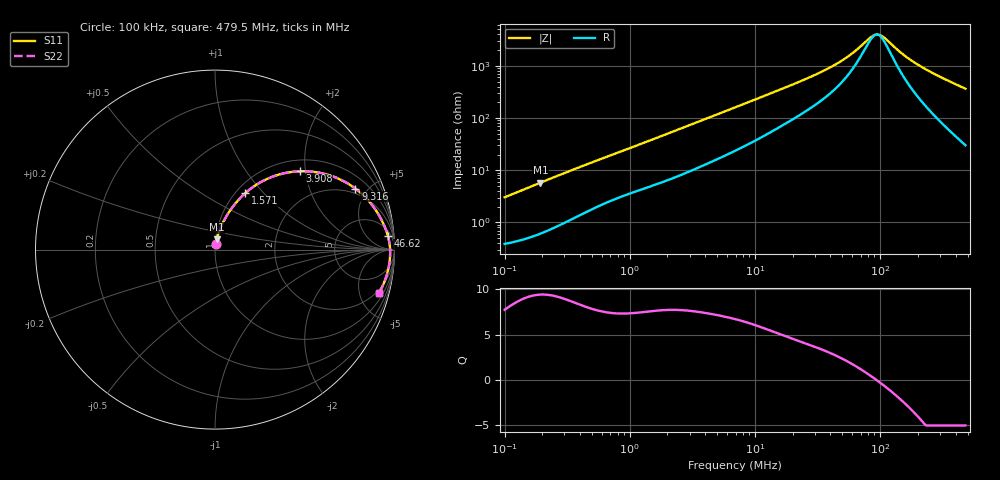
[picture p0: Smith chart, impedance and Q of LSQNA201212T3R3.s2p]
! LSQNA201212T3R3  S-PARAMETER MODEL  ( General Type )
! Model Generated by TAIYO YUDEN Corporation (http://www.ty-top.com)
! Version 2.0
! TAIYO YUDEN Control No. 100810NF25SB-FKC
! Copyright(c) 2007 TAIYO YUDEN CO.,LTD. All Rights Reserved.
! Product Description (link to TY-COMPAS)
! https://ds.yuden.co.jp/TYCOMPAS/or/detail?pn=LSQNA201212T3R3M&u=M
! Products Name : Inductors
! Characteristics :
!  Inductance : 3.3 uH , SRF(min) : 55 MHz , DC Resistance(max) : 0.39 Ohm
!  Rated Current : Saturation :330 mA , Temp Rise : 650 mA (40 degC)
!  Case Size : 2.0 x 1.25 / 0.079 x 0.049 [mm/inch] , Thickness : 1.25 / 0.049 [mm/inch]
!  (Conditions: Temperature = 25 degC , DC Bias Current/Voltage = 0A / 0V)
! External Node Assignments :
!  1  o---GGG---o  2
! GND o---------o GND
! Frequency Range : 0.1MHz  -  479.524407MHz  [ 402 STEP ]
# MHz S RI R 50
! Freq[MHz].  S11 Real  S11 Imag  S21 Real  S21 Imag  S12 Real  S12 Imag  S22 Real  S22 Imag
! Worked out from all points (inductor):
!   401 points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, 100 kHz to 479.5 MHz, reference 50 ohm
!   read as one part in series: L = 4.77 uH near 104.3 kHz
!   highest Q = 9.43 at 192.9 kHz (marker M1), where L = 4.73 uH
!   self-resonance near 93.8 MHz
!   S11 on the Smith chart (normalised r, x): 100 kHz: 1.01, +0.06; 1.571 MHz: 1.10, +0.80; 3.908 MHz: 1.25, +1.86; 9.316 MHz: 1.67, +4.17; 46.62 MHz: 9, +22; 479.5 MHz: 1.60, -7.30
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0.1  0.00475 0.0298  0.9952 -0.0298  0.9952 -0.0298  0.00475 0.0298
0.192869  0.00927 0.0565  0.9907 -0.0565  0.9907 -0.0565  0.00927 0.0565
0.413557  0.0274 0.1135  0.9726 -0.1135  0.9726 -0.1135  0.0274 0.1135
0.886765  0.0793 0.2105  0.9207 -0.2105  0.9207 -0.2105  0.0793 0.2105
1.571316  0.1683 0.3143  0.8317 -0.3143  0.8317 -0.3143  0.1683 0.3143
1.710297  0.1878 0.3308  0.8122 -0.3308  0.8122 -0.3308  0.1878 0.3308
2.725939  0.3298 0.4096  0.6702 -0.4096  0.6702 -0.4096  0.3298 0.4096
3.907965  0.4712 0.4364  0.5288 -0.4364  0.5288 -0.4364  0.4712 0.4364
7.073061  0.7004 0.3895  0.2996 -0.3895  0.2996 -0.3895  0.7004 0.3895
9.316091  0.7825 0.3398  0.2175 -0.3398  0.2175 -0.3398  0.7825 0.3398
15.4911  0.8822 0.239  0.1178 -0.239  0.1178 -0.239  0.8822 0.239
28.6379  0.9411 0.1376  0.0589 -0.1376  0.0589 -0.1376  0.9411 0.1376
46.62166  0.9636 0.0752  0.0364 -0.0752  0.0364 -0.0752  0.9636 0.0752
60.11905  0.9702 0.0467  0.0298 -0.0467  0.0298 -0.0467  0.9702 0.0467
82.61188  0.9747 0.0132  0.0253 -0.0132  0.0253 -0.0132  0.9747 0.0132
89.91882  0.9754 0.0044  0.0246 -0.0044  0.0246 -0.0044  0.9754 0.0044
102.1087  0.9759 -0.00887  0.0241 0.00887  0.0241 0.00887  0.9759 -0.00887
118.4342  0.9759 -0.0246  0.0241 0.0246  0.0241 0.0246  0.9759 -0.0246
152.7219  0.9743 -0.0532  0.0257 0.0532  0.0257 0.0532  0.9743 -0.0532
205.4611  0.9692 -0.0908  0.0308 0.0908  0.0308 0.0908  0.9692 -0.0908
307.304  0.9533 -0.1532  0.0467 0.1532  0.0467 0.1532  0.9533 -0.1532
479.5244  0.9132 -0.2431  0.0868 0.2431  0.0868 0.2431  0.9132 -0.2431
